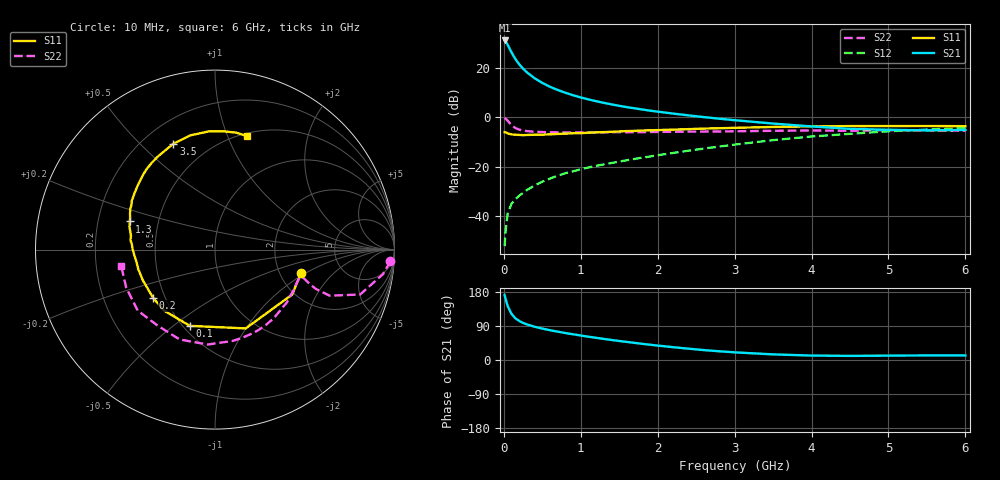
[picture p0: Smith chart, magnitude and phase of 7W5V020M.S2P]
! Infineon Technologies  Discrete & RF Semiconductors
! BFS17W
! Si NPN RF Bipolar Junction Transistor in SOT323
! VCE = 5 V  IC = 20 mA
! Common Emitter S-Parameters:  August  1999
# GHz  S  MA  R  50
!  f  S11  S21  S12  S22
! GHz  MAG  ANG  MAG  ANG  MAG  ANG  MAG  ANG
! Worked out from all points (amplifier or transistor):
!   36 points, 10 MHz to 6 GHz, reference 50 ohm
!   highest |S21| = 30.9 dB at 10 MHz (marker M1)
!   |S21| within 3 dB of that: start of sweep to 70.26 MHz
!   unconditionally stable (mu >= 1): 286.1 MHz to 2.152 GHz; 5.223 GHz to end of sweep
!   at 250 MHz: K = 0.97, MSG = 25.0 dB, |S12| = -30.5 dB
!   at 1.4 GHz: K = 1.16, MAG = 9.4 dB, |S12| = -18.5 dB
!   at 6 GHz: K = 1.05, MAG = -1.7 dB, |S12| = -4.4 dB
!   S11 on the Smith chart (normalised r, x): 10 MHz: 2.61, -0.91; 100 MHz: 0.54, -0.57; 200 MHz: 0.43, -0.29; 1.3 GHz: 0.34, +0.14; 3.5 GHz: 0.32, +0.63; 6 GHz: 0.53, +1.17
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0.01  0.4971 -15.3  35.18 171.6  0.0025 78.7  0.9795 -3.8
0.02  0.4974 -30.3  34.15 163.1  0.0046 78.0  0.946 -8.3
0.05  0.4713 -68.7  28.78 142.4  0.0116 69.5  0.8465 -17.2
0.1  0.4475 -108.3  20.14 121.6  0.0179 58.9  0.688 -21.9
0.15  0.4424 -129.8  14.86 110.0  0.0221 58.5  0.6028 -21.3
0.2  0.4375 -142.1  11.64 103.0  0.0262 61.8  0.5607 -19.9
0.25  0.4334 -150.9  9.496 97.9  0.0297 61.7  0.5359 -18.7
0.3  0.437 -156.8  8.002 93.9  0.034 64.3  0.523 -18.0
0.4  0.4412 -165.9  6.086 87.7  0.0419 66.3  0.5061 -17.6
0.5  0.4435 -171.5  4.898 82.9  0.05 67.9  0.5003 -17.9
0.6  0.4504 -176.0  4.087 78.6  0.0578 69.2  0.4961 -18.9
0.7  0.4582 -179.7  3.529 74.8  0.066 70.1  0.4934 -20.2
0.9  0.4741 173.6  2.761 67.9  0.0808 71.0  0.4909 -23.6
1.1  0.4853 167.2  2.277 61.4  0.0965 71.3  0.4927 -27.7
1.3  0.5002 161.7  1.942 55.6  0.1117 71.9  0.4924 -32.4
1.7  0.5273 152.1  1.506 45.2  0.1439 72.7  0.4967 -42.2
2.2  0.56 140.2  1.18 33.8  0.1896 73.0  0.5066 -55.8
2.8  0.5977 126.4  0.93 23.0  0.2552 70.7  0.5143 -73.2
3.5  0.6343 111.4  0.742 14.8  0.3438 65.0  0.5304 -94.4
4.5  0.6596 93.0  0.58 10.8  0.4605 52.2  0.5305 -127.1
5.5  0.6623 79.7  0.541 12.1  0.5622 39.1  0.5382 -156.8
6  0.6569 74.4  0.551 12.0  0.6025 32.8  0.5302 -169.9
